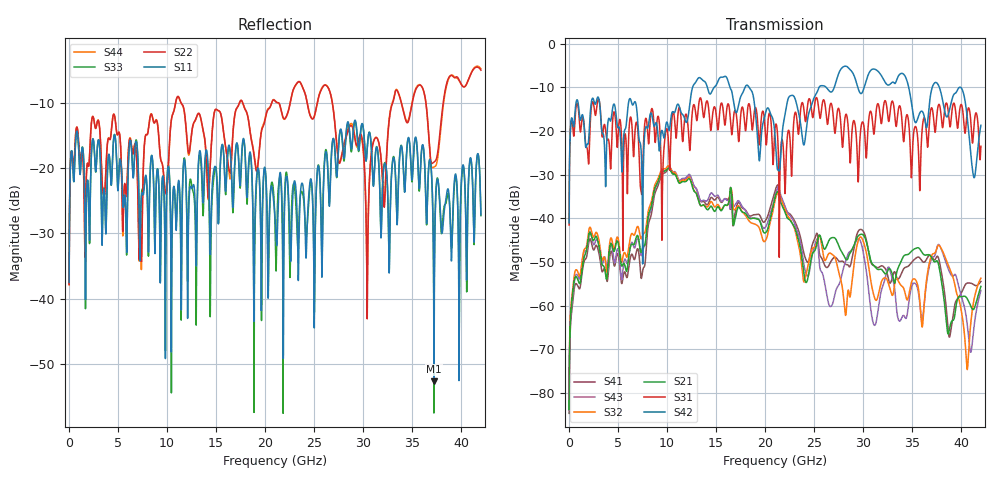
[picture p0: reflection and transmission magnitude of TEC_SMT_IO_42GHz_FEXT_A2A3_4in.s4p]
!! CHANNEL DESCRIPTION: Next Generation 28Gbps High Density SMT I/O Connector
!!  with 4" 5-6-5 Megatron 6 Stripline trace on host side and 1.25" 7-5-7 Megtron 6 Microstrip trace on plug side at 14GHz
!! HOST PCB DESCRIPTION: PCB thickness 2.86 mm, Nelco 4000-13SI (Dk 3.32, Df 0.010)
!!  23 Layer Board, 12 GND planes, 2 Layer route-out on Layers 10,12, 8 mil stub on vias
!!  Pairs on following layers
!!  Layer 10 - A2A3
!! CONNECTOR DESCRIPTION:  Next Generation 28Gbps High Density SMT I/O Connector
!! PLUG-IN CARD DESCRIPTION:  PCB thickness 1mm thick, Nelco 4000-13SI (Dk 3.32, Df 0.010)
!!  6 Layer Board, 4 GND planes, 0.35 x 1.4mm mating pads
!!  Micro-strip diff traces referenced to GND plane 3mils down, 2nd GND plane 15mils from top of board
!!  PCB GND planes are symmetric
!! MODEL DESCRIPTION: TE Connectivity S-parameter model produced from Macro-model
!! MODEL DATE: 9/25/2014 CR1a_GC1i, VR6&12_4
!! MODEL STATUS: Developmental
!! MODEL GEOMETRY: 2 Rows - Rows A, B. 3 pairs in each row, 6 total pairs
!! MODEL FREQUENCY RANGE: DC to 42 GHz in 10 MHz frequency steps
!! MODEL EDGE RATE LIMITATION: 11.90 ps (Using conservative 0.5/Fmax rule of thumb)
!! TIME-DOMAIN TRANSFORM CAUTIONS:
!! 1.) Do not simulate transient edge rates faster than the number listed above.  Edge
!!  rates faster than this number contain significant spectral content at frequencies
!!  above the model's highest frequency.
!! 2.) Even when simulating edge rates that are slower than the number listed above, be
!!  aware that the best time resolution possible with a direct iFFT is (1 / 2Fmax).
!!  As a result, time resolution is typically not adequate for most time-domain
!!  simulations unless tricks such as frequency-domain zero-padding and windowing are
!!  used to minimize leakage and aliasing.
!! 3.) Because the model has a uniform frequency step, a direct iFFT will result in an
!!  impulse that that has a time length given by either (1 / Fstep) or (1 / 2Fstep),
!!  depending on the transform being used.  Care has been taken in selecting the
!!  frequency step to ensure a settled impulse response for the model.  Therefore,
!!  convolution with the model's impulse response should present no issues.  However,
!!  if directly concatenating s-parameter models in the frequency domain a user must
!!  either interpolate necessary interim frequencies or complete impulse response
!!  zero-padding.  Impulse response zero-padding is more difficult, but more accurate.
!! PORT DEFINITIONS:
!! Port  1  ----->  Host, Bot Row  A2  B5  Module, Top Row  <-----  Port  2
!! Port  3  ----->  Host, Bot Row  A3  B6  Module, Top Row  <-----  Port  4
# Hz S MA R 50
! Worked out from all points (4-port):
!   4200 points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, 10 MHz to 42 GHz, reference 50 ohm
!   strongest paths, dB at 10 MHz, 10.51 GHz, 21.01 GHz, 31.51 GHz, 42 GHz:
!     S42: -41.1, -15.7, -21.2, -6.3, -18.7
!     S31: -41.5, -16.8, -19.4, -13.8, -23.5
!     S21: -83.8, -29.7, -35.2, -51.7, -55.6
!     S32: -83.1, -29.3, -35.9, -57.8, -53.7
!     S43: -83.9, -29.2, -35.0, -61.2, -56.5
!     S41: -84.7, -29.6, -33.7, -51.3, -54.5
!   lowest |S11| = -52.7 dB at 37.22 GHz (marker M1), VSWR 1.00, Z = 50.2 - j0.151 ohm
!   |S11| at or under -10 dB: start of sweep to end of sweep
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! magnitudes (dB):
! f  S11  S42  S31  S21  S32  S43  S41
! 10 MHz  -37.5  -41.1  -41.5  -83.8  -83.1  -83.9  -84.7
! 2.1 GHz  -30.8  -18.3  -22.0  -43.2  -42.1  -43.3  -44.8
! 10.14 GHz  -19.8  -19.4  -22.6  -28.5  -28.0  -28.1  -28.6
! 31.14 GHz  -20.6  -5.8  -20.1  -51.0  -58.1  -64.5  -50.9
! 37.22 GHz  -52.7  -9.1  -18.2  -49.9  -48.1  -48.8  -49.5
! 40.59 GHz  -32.1  -16.5  -16.1  -58.4  -74.6  -64.0  -54.9
! 42 GHz  -27.2  -18.7  -23.5  -55.6  -53.7  -56.5  -54.5
